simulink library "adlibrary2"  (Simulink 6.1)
undefined symbols (not defined in the file or in its folder): adlibrary2, ADM, Bit, Black, Box, d2sram_config, DDR, ddr32_config, ddr32xp_config, Generation, II, Inactive, Location, Lower, SDRAM, Simulation, Subsystem, Width, xbsIndex_r3, XPL, XRC, XRM, zbt32_config, zbt64_config, zbtXRC4_config
libraries: xbsIndex_r3 x786
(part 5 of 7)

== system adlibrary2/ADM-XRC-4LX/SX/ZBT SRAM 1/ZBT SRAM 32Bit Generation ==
  d : Inport  Port=1  LatchInput=off
  a : Inport  Port=2  LatchInput=off
  w : Inport  Port=3  LatchInput=off
  r : Inport  Port=4  LatchInput=off
  be : Inport  Port=5  LatchInput=off
  adlocb_in : Inport  Port=6  LatchInput=off
  Black Box : S-Function  FunctionName=xlblackbox2  Parameters=sfcn_mwsv__  mask(Xilinx Blackbox Block){init_code=zbtXRC4_config, sim_method=Inactive, engine_block=, show_param=on, xl_area=[88, 129, 0, 35, 0, 0, 0], xl_use_area=on, adlocb_devid=1}
      mask prompts: init_code "Block Configuration M-Function"; sim_method "Simulation Mode"; engine_block "HDL Co-Simulator To Use  (specify helper block by name)"; show_param "---------------------- Show Implementation Parameters -----------------------------------------------------------------------------------"; xl_area "FPGA Area [Slices, FFs, BRAMs, LUTs, IOBs, Emb. Mults, TBUFs]"; xl_use_area "Use Area Above For Estimation"; adlocb_devid "ADLOCB DEV ID"
      mask help: Incorporates black box HDL and simulation model into a System Generator design. You must supply a Black Box with certain information about the HDL component you would like to bring into System Generator. This information is provided through a Matlab function. When "Simulation Mode" is set to "Inactive," you will typically want to provide a separate simulation model by using a Simulation Multiplexer. When "Simulation Mode" is set to "Use HDL Co-Simulation", you must include a ModelSim block in the design.
      mask init:
      | [designRoot, family, part, speed, package, simulinkPeriod, sysclkPeriod, dbl_ovrd, trimVbit] = xlSysgenSettings(gcb,0,0);
      | 
      | [bg,fg] = xlcmap('XBlock');
      | iPos = get_param(gcb,'Position');
      | iWidth=iPos(3)-iPos(1); iHeight=iPos(4)-iPos(2);
      | iCx=iWidth/2;
      | iCy=iHeight/2;
      | [logoX, logoY] = xlogo(iPos);
      | zstr='z'; zpstr='-1';
      | zstrx = iCx-3; if (zstrx<16) zstr='';zpstr=''; end
      | zstry = iCy;
      | 
      | precision0 = 1;
      | latency = 0;
      | dblOvrd = 0;
      | 
      | mdlPath = xlGetMdlDir(bdroot);
      | 
      | refBlk = get_param(gcb,'referenceBlock');
      | if (isempty(refBlk) | strncmp(refBlk,'xbsIndex',8))
      | 	srcPath = mdlPath;
      | else
      | 	srcPath = xlPathToReference;
      | 	if (isempty(srcPath))
      | 		srcPath = mdlPath;
      | 	end
      | end
      | 
      | if (sim_method==2)
      | 	validEngineBlock = 0;
      | 	try
      | 	  engineBlock = xlBlockNameRelPath(get_param(gcb,'Parent'),engine_block);
      | 	catch
      | 	  engineBlock = '//';
      | 	end
      | 	try 
      | 	  engineWorkDir = get_param(engineBlock,'dir');
      | 	  validEngineBlock = 1;
      | 	catch
      | 	end
      | end
      | 
      | % just pass everything to s-function
      | sfcn_mwsv__ = get_param(gcb, 'MaskWSVariables');
      | adlocb_devid = 1;
      | plabel = xlbbPortLabelStruct(gcb,init_code,mdlPath);
  Constant : Constant  Value=0
  Terminator{,1..3} (4 alike) : Terminator
  ra1 : xbsIndex_r3/Gateway Out  output_type=Double  nbits=8  bin_pt=6  arith_type=Boolean  quantization=Truncate  overflow=Wrap  hdl_port=on  timing_constraint=None  locs_specified=off  LOCs={}  needs_fixed_name=off  show_param=off
  rc1 : xbsIndex_r3/Gateway Out  output_type=Double  nbits=8  bin_pt=6  arith_type=Boolean  quantization=Truncate  overflow=Wrap  hdl_port=on  timing_constraint=None  locs_specified=off  LOCs={}  needs_fixed_name=off  show_param=off
  rd1_i : xbsIndex_r3/Gateway In  arith_type=Unsigned  n_bits=32  bin_pt=0  quantization=Truncate  overflow=Wrap  period=1  timing_constraint=None  locs_specified=off  LOCs={}  needs_fixed_name=off  dbl_ovrd=off  show_param=off
  rd1_o : xbsIndex_r3/Gateway Out  output_type=Double  nbits=8  bin_pt=6  arith_type=Boolean  quantization=Truncate  overflow=Wrap  hdl_port=on  timing_constraint=None  locs_specified=off  LOCs={}  needs_fixed_name=off  show_param=off
  rd1_t : xbsIndex_r3/Gateway Out  output_type=Double  nbits=8  bin_pt=6  arith_type=Boolean  quantization=Truncate  overflow=Wrap  hdl_port=on  timing_constraint=None  locs_specified=off  LOCs={}  needs_fixed_name=off  show_param=off
  q : Outport
  qv : Outport  Port=2
  adlocb_out : Outport  Port=3
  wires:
  Black Box/7 -> adlocb_out/1
  adlocb_in/1 -> Black Box/7
  be/1 -> Black Box/5
  rd1_i/1 -> Black Box/6
  d/1 -> Black Box/1
  Black Box/1 -> q/1
  Black Box/2 -> qv/1
  Constant/1 -> rd1_i/1
  rd1_o/1 -> Terminator/1
  rd1_t/1 -> Terminator1/1
  ra1/1 -> Terminator2/1
  rc1/1 -> Terminator3/1
  a/1 -> Black Box/2
  w/1 -> Black Box/3
  r/1 -> Black Box/4
  Black Box/3 -> rd1_o/1
  Black Box/4 -> rd1_t/1
  Black Box/5 -> ra1/1
  Black Box/6 -> rc1/1

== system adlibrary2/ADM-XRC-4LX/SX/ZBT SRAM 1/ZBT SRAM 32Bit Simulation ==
  d : Inport  Port=1  LatchInput=off
  a : Inport  Port=2  LatchInput=off
  w : Inport  Port=3  LatchInput=off
  r : Inport  Port=4  LatchInput=off
  be : Inport  Port=5  LatchInput=off
  Disregard Subsystem : xbsIndex_r3/Disregard Subsystem  Tag=discardX
  Gateway In6 : xbsIndex_r3/Gateway In  arith_type=Boolean  n_bits=1  bin_pt=0  quantization=Truncate  overflow=Wrap  period=1  timing_constraint=None  locs_specified=off  LOCs={}  needs_fixed_name=off  dbl_ovrd=on  show_param=off
  Gateway In7 : xbsIndex_r3/Gateway In  arith_type=Unsigned  n_bits=32  bin_pt=0  quantization=Truncate  overflow=Wrap  period=1  timing_constraint=None  locs_specified=off  LOCs={}  needs_fixed_name=off  dbl_ovrd=on  show_param=off
  Gateway Out{,1..4} (5 alike) : xbsIndex_r3/Gateway Out  output_type=Double  nbits=8  bin_pt=6  arith_type=Boolean  quantization=Truncate  overflow=Wrap  hdl_port=off  timing_constraint=None  locs_specified=off  LOCs={}  needs_fixed_name=off  show_param=off
  S-Function : S-Function  FunctionName=zbt32  Parameters=1
  q : Outport
  qv : Outport  Port=2
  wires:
  be/1 -> Gateway Out4/1
  Gateway Out4/1 -> S-Function/5
  d/1 -> Gateway Out/1
  a/1 -> Gateway Out1/1
  w/1 -> Gateway Out2/1
  r/1 -> Gateway Out3/1
  S-Function/1 -> Gateway In7/1
  Gateway Out/1 -> S-Function/1
  Gateway Out1/1 -> S-Function/2
  Gateway Out2/1 -> S-Function/3
  Gateway Out3/1 -> S-Function/4
  Gateway In6/1 -> qv/1
  Gateway In7/1 -> q/1
  S-Function/2 -> Gateway In6/1

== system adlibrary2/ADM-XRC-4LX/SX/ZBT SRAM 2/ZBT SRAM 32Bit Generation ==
  d : Inport  Port=1  LatchInput=off
  a : Inport  Port=2  LatchInput=off
  w : Inport  Port=3  LatchInput=off
  r : Inport  Port=4  LatchInput=off
  be : Inport  Port=5  LatchInput=off
  adlocb_in : Inport  Port=6  LatchInput=off
  Black Box : S-Function  FunctionName=xlblackbox2  Parameters=sfcn_mwsv__  mask(Xilinx Blackbox Block){init_code=zbtXRC4_config, sim_method=Inactive, engine_block=, show_param=on, xl_area=[88, 129, 0, 35, 0, 0, 0], xl_use_area=on, adlocb_devid=2}
      mask prompts: init_code "Block Configuration M-Function"; sim_method "Simulation Mode"; engine_block "HDL Co-Simulator To Use  (specify helper block by name)"; show_param "---------------------- Show Implementation Parameters -----------------------------------------------------------------------------------"; xl_area "FPGA Area [Slices, FFs, BRAMs, LUTs, IOBs, Emb. Mults, TBUFs]"; xl_use_area "Use Area Above For Estimation"; adlocb_devid "ADLOCB DEV ID"
      mask help: Incorporates black box HDL and simulation model into a System Generator design. You must supply a Black Box with certain information about the HDL component you would like to bring into System Generator. This information is provided through a Matlab function. When "Simulation Mode" is set to "Inactive," you will typically want to provide a separate simulation model by using a Simulation Multiplexer. When "Simulation Mode" is set to "Use HDL Co-Simulation", you must include a ModelSim block in the design.
      mask init:
      | [designRoot, family, part, speed, package, simulinkPeriod, sysclkPeriod, dbl_ovrd, trimVbit] = xlSysgenSettings(gcb,0,0);
      | 
      | [bg,fg] = xlcmap('XBlock');
      | iPos = get_param(gcb,'Position');
      | iWidth=iPos(3)-iPos(1); iHeight=iPos(4)-iPos(2);
      | iCx=iWidth/2;
      | iCy=iHeight/2;
      | [logoX, logoY] = xlogo(iPos);
      | zstr='z'; zpstr='-1';
      | zstrx = iCx-3; if (zstrx<16) zstr='';zpstr=''; end
      | zstry = iCy;
      | 
      | precision0 = 1;
      | latency = 0;
      | dblOvrd = 0;
      | 
      | mdlPath = xlGetMdlDir(bdroot);
      | 
      | refBlk = get_param(gcb,'referenceBlock');
      | if (isempty(refBlk) | strncmp(refBlk,'xbsIndex',8))
      | 	srcPath = mdlPath;
      | else
      | 	srcPath = xlPathToReference;
      | 	if (isempty(srcPath))
      | 		srcPath = mdlPath;
      | 	end
      | end
      | 
      | if (sim_method==2)
      | 	validEngineBlock = 0;
      | 	try
      | 	  engineBlock = xlBlockNameRelPath(get_param(gcb,'Parent'),engine_block);
      | 	catch
      | 	  engineBlock = '//';
      | 	end
      | 	try 
      | 	  engineWorkDir = get_param(engineBlock,'dir');
      | 	  validEngineBlock = 1;
      | 	catch
      | 	end
      | end
      | 
      | % just pass everything to s-function
      | sfcn_mwsv__ = get_param(gcb, 'MaskWSVariables');
      | 
      | plabel = xlbbPortLabelStruct(gcb,init_code,mdlPath);
  Constant : Constant  Value=0
  Terminator{,1..3} (4 alike) : Terminator
  ra2 : xbsIndex_r3/Gateway Out  output_type=Double  nbits=8  bin_pt=6  arith_type=Boolean  quantization=Truncate  overflow=Wrap  hdl_port=on  timing_constraint=None  locs_specified=off  LOCs={}  needs_fixed_name=off  show_param=off
  rc2 : xbsIndex_r3/Gateway Out  output_type=Double  nbits=8  bin_pt=6  arith_type=Boolean  quantization=Truncate  overflow=Wrap  hdl_port=on  timing_constraint=None  locs_specified=off  LOCs={}  needs_fixed_name=off  show_param=off
  rd2_i : xbsIndex_r3/Gateway In  arith_type=Unsigned  n_bits=32  bin_pt=0  quantization=Truncate  overflow=Wrap  period=1  timing_constraint=None  locs_specified=off  LOCs={}  needs_fixed_name=off  dbl_ovrd=off  show_param=off
  rd2_o : xbsIndex_r3/Gateway Out  output_type=Double  nbits=8  bin_pt=6  arith_type=Boolean  quantization=Truncate  overflow=Wrap  hdl_port=on  timing_constraint=None  locs_specified=off  LOCs={}  needs_fixed_name=off  show_param=off
  rd2_t : xbsIndex_r3/Gateway Out  output_type=Double  nbits=8  bin_pt=6  arith_type=Boolean  quantization=Truncate  overflow=Wrap  hdl_port=on  timing_constraint=None  locs_specified=off  LOCs={}  needs_fixed_name=off  show_param=off
  q : Outport
  qv : Outport  Port=2
  adlocb_out : Outport  Port=3
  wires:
  Black Box/7 -> adlocb_out/1
  adlocb_in/1 -> Black Box/7
  be/1 -> Black Box/5
  rd2_i/1 -> Black Box/6
  d/1 -> Black Box/1
  Black Box/1 -> q/1
  Black Box/2 -> qv/1
  Constant/1 -> rd2_i/1
  rd2_o/1 -> Terminator/1
  rd2_t/1 -> Terminator1/1
  ra2/1 -> Terminator2/1
  rc2/1 -> Terminator3/1
  a/1 -> Black Box/2
  w/1 -> Black Box/3
  r/1 -> Black Box/4
  Black Box/3 -> rd2_o/1
  Black Box/4 -> rd2_t/1
  Black Box/5 -> ra2/1
  Black Box/6 -> rc2/1

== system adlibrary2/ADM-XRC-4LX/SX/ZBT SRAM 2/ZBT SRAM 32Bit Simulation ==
  d : Inport  Port=1  LatchInput=off
  a : Inport  Port=2  LatchInput=off
  w : Inport  Port=3  LatchInput=off
  r : Inport  Port=4  LatchInput=off
  be : Inport  Port=5  LatchInput=off
  Disregard Subsystem : xbsIndex_r3/Disregard Subsystem  Tag=discardX
  Gateway In6 : xbsIndex_r3/Gateway In  arith_type=Boolean  n_bits=1  bin_pt=0  quantization=Truncate  overflow=Wrap  period=1  timing_constraint=None  locs_specified=off  LOCs={}  needs_fixed_name=off  dbl_ovrd=on  show_param=off
  Gateway In7 : xbsIndex_r3/Gateway In  arith_type=Unsigned  n_bits=32  bin_pt=0  quantization=Truncate  overflow=Wrap  period=1  timing_constraint=None  locs_specified=off  LOCs={}  needs_fixed_name=off  dbl_ovrd=on  show_param=off
  Gateway Out{,1..4} (5 alike) : xbsIndex_r3/Gateway Out  output_type=Double  nbits=8  bin_pt=6  arith_type=Boolean  quantization=Truncate  overflow=Wrap  hdl_port=off  timing_constraint=None  locs_specified=off  LOCs={}  needs_fixed_name=off  show_param=off
  S-Function : S-Function  FunctionName=zbt32  Parameters=2
  q : Outport
  qv : Outport  Port=2
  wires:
  be/1 -> Gateway Out4/1
  Gateway Out4/1 -> S-Function/5
  d/1 -> Gateway Out/1
  a/1 -> Gateway Out1/1
  w/1 -> Gateway Out2/1
  r/1 -> Gateway Out3/1
  S-Function/1 -> Gateway In7/1
  Gateway Out/1 -> S-Function/1
  Gateway Out1/1 -> S-Function/2
  Gateway Out2/1 -> S-Function/3
  Gateway Out3/1 -> S-Function/4
  Gateway In6/1 -> qv/1
  Gateway In7/1 -> q/1
  S-Function/2 -> Gateway In6/1

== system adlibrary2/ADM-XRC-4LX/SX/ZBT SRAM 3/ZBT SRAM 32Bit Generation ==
  d : Inport  Port=1  LatchInput=off
  a : Inport  Port=2  LatchInput=off
  w : Inport  Port=3  LatchInput=off
  r : Inport  Port=4  LatchInput=off
  be : Inport  Port=5  LatchInput=off
  adlocb_in : Inport  Port=6  LatchInput=off
  Black Box : S-Function  FunctionName=xlblackbox2  Parameters=sfcn_mwsv__  mask(Xilinx Blackbox Block){init_code=zbtXRC4_config, sim_method=Inactive, engine_block=, show_param=on, xl_area=[88, 129, 0, 35, 0, 0, 0], xl_use_area=on, adlocb_devid=3}
      mask prompts: init_code "Block Configuration M-Function"; sim_method "Simulation Mode"; engine_block "HDL Co-Simulator To Use  (specify helper block by name)"; show_param "---------------------- Show Implementation Parameters -----------------------------------------------------------------------------------"; xl_area "FPGA Area [Slices, FFs, BRAMs, LUTs, IOBs, Emb. Mults, TBUFs]"; xl_use_area "Use Area Above For Estimation"; adlocb_devid "ADLOCB DEV ID"
      mask help: Incorporates black box HDL and simulation model into a System Generator design. You must supply a Black Box with certain information about the HDL component you would like to bring into System Generator. This information is provided through a Matlab function. When "Simulation Mode" is set to "Inactive," you will typically want to provide a separate simulation model by using a Simulation Multiplexer. When "Simulation Mode" is set to "Use HDL Co-Simulation", you must include a ModelSim block in the design.
      mask init:
      | [designRoot, family, part, speed, package, simulinkPeriod, sysclkPeriod, dbl_ovrd, trimVbit] = xlSysgenSettings(gcb,0,0);
      | 
      | [bg,fg] = xlcmap('XBlock');
      | iPos = get_param(gcb,'Position');
      | iWidth=iPos(3)-iPos(1); iHeight=iPos(4)-iPos(2);
      | iCx=iWidth/2;
      | iCy=iHeight/2;
      | [logoX, logoY] = xlogo(iPos);
      | zstr='z'; zpstr='-1';
      | zstrx = iCx-3; if (zstrx<16) zstr='';zpstr=''; end
      | zstry = iCy;
      | 
      | precision0 = 1;
      | latency = 0;
      | dblOvrd = 0;
      | 
      | mdlPath = xlGetMdlDir(bdroot);
      | 
      | refBlk = get_param(gcb,'referenceBlock');
      | if (isempty(refBlk) | strncmp(refBlk,'xbsIndex',8))
      | 	srcPath = mdlPath;
      | else
      | 	srcPath = xlPathToReference;
      | 	if (isempty(srcPath))
      | 		srcPath = mdlPath;
      | 	end
      | end
      | 
      | if (sim_method==2)
      | 	validEngineBlock = 0;
      | 	try
      | 	  engineBlock = xlBlockNameRelPath(get_param(gcb,'Parent'),engine_block);
      | 	catch
      | 	  engineBlock = '//';
      | 	end
      | 	try 
      | 	  engineWorkDir = get_param(engineBlock,'dir');
      | 	  validEngineBlock = 1;
      | 	catch
      | 	end
      | end
      | 
      | % just pass everything to s-function
      | sfcn_mwsv__ = get_param(gcb, 'MaskWSVariables');
      | adlocb_devid = 1;
      | plabel = xlbbPortLabelStruct(gcb,init_code,mdlPath);
  Constant : Constant  Value=0
  Terminator{,1..3} (4 alike) : Terminator
  ra3 : xbsIndex_r3/Gateway Out  output_type=Double  nbits=8  bin_pt=6  arith_type=Boolean  quantization=Truncate  overflow=Wrap  hdl_port=on  timing_constraint=None  locs_specified=off  LOCs={}  needs_fixed_name=off  show_param=off
  rc3 : xbsIndex_r3/Gateway Out  output_type=Double  nbits=8  bin_pt=6  arith_type=Boolean  quantization=Truncate  overflow=Wrap  hdl_port=on  timing_constraint=None  locs_specified=off  LOCs={}  needs_fixed_name=off  show_param=off
  rd3_i : xbsIndex_r3/Gateway In  arith_type=Unsigned  n_bits=32  bin_pt=0  quantization=Truncate  overflow=Wrap  period=1  timing_constraint=None  locs_specified=off  LOCs={}  needs_fixed_name=off  dbl_ovrd=off  show_param=off
  rd3_o : xbsIndex_r3/Gateway Out  output_type=Double  nbits=8  bin_pt=6  arith_type=Boolean  quantization=Truncate  overflow=Wrap  hdl_port=on  timing_constraint=None  locs_specified=off  LOCs={}  needs_fixed_name=off  show_param=off
  rd3_t : xbsIndex_r3/Gateway Out  output_type=Double  nbits=8  bin_pt=6  arith_type=Boolean  quantization=Truncate  overflow=Wrap  hdl_port=on  timing_constraint=None  locs_specified=off  LOCs={}  needs_fixed_name=off  show_param=off
  q : Outport
  qv : Outport  Port=2
  adlocb_out : Outport  Port=3
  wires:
  Black Box/6 -> rc3/1
  Black Box/5 -> ra3/1
  Black Box/4 -> rd3_t/1
  Black Box/3 -> rd3_o/1
  r/1 -> Black Box/4
  w/1 -> Black Box/3
  a/1 -> Black Box/2
  rc3/1 -> Terminator3/1
  ra3/1 -> Terminator2/1
  rd3_t/1 -> Terminator1/1
  rd3_o/1 -> Terminator/1
  Constant/1 -> rd3_i/1
  Black Box/2 -> qv/1
  Black Box/1 -> q/1
  d/1 -> Black Box/1
  rd3_i/1 -> Black Box/6
  be/1 -> Black Box/5
  adlocb_in/1 -> Black Box/7
  Black Box/7 -> adlocb_out/1

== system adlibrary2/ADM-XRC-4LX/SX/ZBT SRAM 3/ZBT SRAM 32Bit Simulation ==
  d : Inport  Port=1  LatchInput=off
  a : Inport  Port=2  LatchInput=off
  w : Inport  Port=3  LatchInput=off
  r : Inport  Port=4  LatchInput=off
  be : Inport  Port=5  LatchInput=off
  Disregard Subsystem : xbsIndex_r3/Disregard Subsystem  Tag=discardX
  Gateway In6 : xbsIndex_r3/Gateway In  arith_type=Boolean  n_bits=1  bin_pt=0  quantization=Truncate  overflow=Wrap  period=1  timing_constraint=None  locs_specified=off  LOCs={}  needs_fixed_name=off  dbl_ovrd=on  show_param=off
  Gateway In7 : xbsIndex_r3/Gateway In  arith_type=Unsigned  n_bits=32  bin_pt=0  quantization=Truncate  overflow=Wrap  period=1  timing_constraint=None  locs_specified=off  LOCs={}  needs_fixed_name=off  dbl_ovrd=on  show_param=off
  Gateway Out{,1..4} (5 alike) : xbsIndex_r3/Gateway Out  output_type=Double  nbits=8  bin_pt=6  arith_type=Boolean  quantization=Truncate  overflow=Wrap  hdl_port=off  timing_constraint=None  locs_specified=off  LOCs={}  needs_fixed_name=off  show_param=off
  S-Function : S-Function  FunctionName=zbt32  Parameters=3
  q : Outport
  qv : Outport  Port=2
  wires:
  S-Function/2 -> Gateway In6/1
  Gateway In7/1 -> q/1
  Gateway In6/1 -> qv/1
  Gateway Out3/1 -> S-Function/4
  Gateway Out2/1 -> S-Function/3
  Gateway Out1/1 -> S-Function/2
  Gateway Out/1 -> S-Function/1
  S-Function/1 -> Gateway In7/1
  r/1 -> Gateway Out3/1
  w/1 -> Gateway Out2/1
  a/1 -> Gateway Out1/1
  d/1 -> Gateway Out/1
  Gateway Out4/1 -> S-Function/5
  be/1 -> Gateway Out4/1

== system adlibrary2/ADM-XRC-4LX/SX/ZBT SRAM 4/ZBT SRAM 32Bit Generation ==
  d : Inport  Port=1  LatchInput=off
  a : Inport  Port=2  LatchInput=off
  w : Inport  Port=3  LatchInput=off
  r : Inport  Port=4  LatchInput=off
  be : Inport  Port=5  LatchInput=off
  adlocb_in : Inport  Port=6  LatchInput=off
  Black Box : S-Function  FunctionName=xlblackbox2  Parameters=sfcn_mwsv__  mask(Xilinx Blackbox Block){init_code=zbtXRC4_config, sim_method=Inactive, engine_block=, show_param=on, xl_area=[88, 129, 0, 35, 0, 0, 0], xl_use_area=on, adlocb_devid=4}
      mask prompts: init_code "Block Configuration M-Function"; sim_method "Simulation Mode"; engine_block "HDL Co-Simulator To Use  (specify helper block by name)"; show_param "---------------------- Show Implementation Parameters -----------------------------------------------------------------------------------"; xl_area "FPGA Area [Slices, FFs, BRAMs, LUTs, IOBs, Emb. Mults, TBUFs]"; xl_use_area "Use Area Above For Estimation"; adlocb_devid "ADLOCB DEV ID"
      mask help: Incorporates black box HDL and simulation model into a System Generator design. You must supply a Black Box with certain information about the HDL component you would like to bring into System Generator. This information is provided through a Matlab function. When "Simulation Mode" is set to "Inactive," you will typically want to provide a separate simulation model by using a Simulation Multiplexer. When "Simulation Mode" is set to "Use HDL Co-Simulation", you must include a ModelSim block in the design.
      mask init:
      | [designRoot, family, part, speed, package, simulinkPeriod, sysclkPeriod, dbl_ovrd, trimVbit] = xlSysgenSettings(gcb,0,0);
      | 
      | [bg,fg] = xlcmap('XBlock');
      | iPos = get_param(gcb,'Position');
      | iWidth=iPos(3)-iPos(1); iHeight=iPos(4)-iPos(2);
      | iCx=iWidth/2;
      | iCy=iHeight/2;
      | [logoX, logoY] = xlogo(iPos);
      | zstr='z'; zpstr='-1';
      | zstrx = iCx-3; if (zstrx<16) zstr='';zpstr=''; end
      | zstry = iCy;
      | 
      | precision0 = 1;
      | latency = 0;
      | dblOvrd = 0;
      | 
      | mdlPath = xlGetMdlDir(bdroot);
      | 
      | refBlk = get_param(gcb,'referenceBlock');
      | if (isempty(refBlk) | strncmp(refBlk,'xbsIndex',8))
      | 	srcPath = mdlPath;
      | else
      | 	srcPath = xlPathToReference;
      | 	if (isempty(srcPath))
      | 		srcPath = mdlPath;
      | 	end
      | end
      | 
      | if (sim_method==2)
      | 	validEngineBlock = 0;
      | 	try
      | 	  engineBlock = xlBlockNameRelPath(get_param(gcb,'Parent'),engine_block);
      | 	catch
      | 	  engineBlock = '//';
      | 	end
      | 	try 
      | 	  engineWorkDir = get_param(engineBlock,'dir');
      | 	  validEngineBlock = 1;
      | 	catch
      | 	end
      | end
      | 
      | % just pass everything to s-function
      | sfcn_mwsv__ = get_param(gcb, 'MaskWSVariables');
      | 
      | plabel = xlbbPortLabelStruct(gcb,init_code,mdlPath);
  Constant : Constant  Value=0
  Terminator{,1..3} (4 alike) : Terminator
  ra4 : xbsIndex_r3/Gateway Out  output_type=Double  nbits=8  bin_pt=6  arith_type=Boolean  quantization=Truncate  overflow=Wrap  hdl_port=on  timing_constraint=None  locs_specified=off  LOCs={}  needs_fixed_name=off  show_param=off
  rc4 : xbsIndex_r3/Gateway Out  output_type=Double  nbits=8  bin_pt=6  arith_type=Boolean  quantization=Truncate  overflow=Wrap  hdl_port=on  timing_constraint=None  locs_specified=off  LOCs={}  needs_fixed_name=off  show_param=off
  rd4_i : xbsIndex_r3/Gateway In  arith_type=Unsigned  n_bits=32  bin_pt=0  quantization=Truncate  overflow=Wrap  period=1  timing_constraint=None  locs_specified=off  LOCs={}  needs_fixed_name=off  dbl_ovrd=off  show_param=off
  rd4_o : xbsIndex_r3/Gateway Out  output_type=Double  nbits=8  bin_pt=6  arith_type=Boolean  quantization=Truncate  overflow=Wrap  hdl_port=on  timing_constraint=None  locs_specified=off  LOCs={}  needs_fixed_name=off  show_param=off
  rd4_t : xbsIndex_r3/Gateway Out  output_type=Double  nbits=8  bin_pt=6  arith_type=Boolean  quantization=Truncate  overflow=Wrap  hdl_port=on  timing_constraint=None  locs_specified=off  LOCs={}  needs_fixed_name=off  show_param=off
  q : Outport
  qv : Outport  Port=2
  adlocb_out : Outport  Port=3
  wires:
  Black Box/7 -> adlocb_out/1
  adlocb_in/1 -> Black Box/7
  be/1 -> Black Box/5
  rd4_i/1 -> Black Box/6
  d/1 -> Black Box/1
  Black Box/1 -> q/1
  Black Box/2 -> qv/1
  Constant/1 -> rd4_i/1
  rd4_o/1 -> Terminator/1
  rd4_t/1 -> Terminator1/1
  ra4/1 -> Terminator2/1
  rc4/1 -> Terminator3/1
  a/1 -> Black Box/2
  w/1 -> Black Box/3
  r/1 -> Black Box/4
  Black Box/3 -> rd4_o/1
  Black Box/4 -> rd4_t/1
  Black Box/5 -> ra4/1
  Black Box/6 -> rc4/1

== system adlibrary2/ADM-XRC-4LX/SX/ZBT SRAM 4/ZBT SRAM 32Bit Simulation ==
  d : Inport  Port=1  LatchInput=off
  a : Inport  Port=2  LatchInput=off
  w : Inport  Port=3  LatchInput=off
  r : Inport  Port=4  LatchInput=off
  be : Inport  Port=5  LatchInput=off
  Disregard Subsystem : xbsIndex_r3/Disregard Subsystem  Tag=discardX
  Gateway In6 : xbsIndex_r3/Gateway In  arith_type=Boolean  n_bits=1  bin_pt=0  quantization=Truncate  overflow=Wrap  period=1  timing_constraint=None  locs_specified=off  LOCs={}  needs_fixed_name=off  dbl_ovrd=on  show_param=off
  Gateway In7 : xbsIndex_r3/Gateway In  arith_type=Unsigned  n_bits=32  bin_pt=0  quantization=Truncate  overflow=Wrap  period=1  timing_constraint=None  locs_specified=off  LOCs={}  needs_fixed_name=off  dbl_ovrd=on  show_param=off
  Gateway Out{,1..4} (5 alike) : xbsIndex_r3/Gateway Out  output_type=Double  nbits=8  bin_pt=6  arith_type=Boolean  quantization=Truncate  overflow=Wrap  hdl_port=off  timing_constraint=None  locs_specified=off  LOCs={}  needs_fixed_name=off  show_param=off
  S-Function : S-Function  FunctionName=zbt32  Parameters=4
  q : Outport
  qv : Outport  Port=2
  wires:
  be/1 -> Gateway Out4/1
  Gateway Out4/1 -> S-Function/5
  d/1 -> Gateway Out/1
  a/1 -> Gateway Out1/1
  w/1 -> Gateway Out2/1
  r/1 -> Gateway Out3/1
  S-Function/1 -> Gateway In7/1
  Gateway Out/1 -> S-Function/1
  Gateway Out1/1 -> S-Function/2
  Gateway Out2/1 -> S-Function/3
  Gateway Out3/1 -> S-Function/4
  Gateway In6/1 -> qv/1
  Gateway In7/1 -> q/1
  S-Function/2 -> Gateway In6/1

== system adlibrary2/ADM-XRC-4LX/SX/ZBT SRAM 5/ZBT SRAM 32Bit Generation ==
  d : Inport  Port=1  LatchInput=off
  a : Inport  Port=2  LatchInput=off
  w : Inport  Port=3  LatchInput=off
  r : Inport  Port=4  LatchInput=off
  be : Inport  Port=5  LatchInput=off
  adlocb_in : Inport  Port=6  LatchInput=off
  Black Box : S-Function  FunctionName=xlblackbox2  Parameters=sfcn_mwsv__  mask(Xilinx Blackbox Block){init_code=zbtXRC4_config, sim_method=Inactive, engine_block=, show_param=on, xl_area=[88, 129, 0, 35, 0, 0, 0], xl_use_area=on, adlocb_devid=5}
      mask prompts: init_code "Block Configuration M-Function"; sim_method "Simulation Mode"; engine_block "HDL Co-Simulator To Use  (specify helper block by name)"; show_param "---------------------- Show Implementation Parameters -----------------------------------------------------------------------------------"; xl_area "FPGA Area [Slices, FFs, BRAMs, LUTs, IOBs, Emb. Mults, TBUFs]"; xl_use_area "Use Area Above For Estimation"; adlocb_devid "ADLOCB DEV ID"
      mask help: Incorporates black box HDL and simulation model into a System Generator design. You must supply a Black Box with certain information about the HDL component you would like to bring into System Generator. This information is provided through a Matlab function. When "Simulation Mode" is set to "Inactive," you will typically want to provide a separate simulation model by using a Simulation Multiplexer. When "Simulation Mode" is set to "Use HDL Co-Simulation", you must include a ModelSim block in the design.
      mask init:
      | [designRoot, family, part, speed, package, simulinkPeriod, sysclkPeriod, dbl_ovrd, trimVbit] = xlSysgenSettings(gcb,0,0);
      | 
      | [bg,fg] = xlcmap('XBlock');
      | iPos = get_param(gcb,'Position');
      | iWidth=iPos(3)-iPos(1); iHeight=iPos(4)-iPos(2);
      | iCx=iWidth/2;
      | iCy=iHeight/2;
      | [logoX, logoY] = xlogo(iPos);
      | zstr='z'; zpstr='-1';
      | zstrx = iCx-3; if (zstrx<16) zstr='';zpstr=''; end
      | zstry = iCy;
      | 
      | precision0 = 1;
      | latency = 0;
      | dblOvrd = 0;
      | 
      | mdlPath = xlGetMdlDir(bdroot);
      | 
      | refBlk = get_param(gcb,'referenceBlock');
      | if (isempty(refBlk) | strncmp(refBlk,'xbsIndex',8))
      | 	srcPath = mdlPath;
      | else
      | 	srcPath = xlPathToReference;
      | 	if (isempty(srcPath))
      | 		srcPath = mdlPath;
      | 	end
      | end
      | 
      | if (sim_method==2)
      | 	validEngineBlock = 0;
      | 	try
      | 	  engineBlock = xlBlockNameRelPath(get_param(gcb,'Parent'),engine_block);
      | 	catch
      | 	  engineBlock = '//';
      | 	end
      | 	try 
      | 	  engineWorkDir = get_param(engineBlock,'dir');
      | 	  validEngineBlock = 1;
      | 	catch
      | 	end
      | end
      | 
      | % just pass everything to s-function
      | sfcn_mwsv__ = get_param(gcb, 'MaskWSVariables');
      | adlocb_devid = 1;
      | plabel = xlbbPortLabelStruct(gcb,init_code,mdlPath);
  Constant : Constant  Value=0
  Terminator{,1..3} (4 alike) : Terminator
  ra5 : xbsIndex_r3/Gateway Out  output_type=Double  nbits=8  bin_pt=6  arith_type=Boolean  quantization=Truncate  overflow=Wrap  hdl_port=on  timing_constraint=None  locs_specified=off  LOCs={}  needs_fixed_name=off  show_param=off
  rc5 : xbsIndex_r3/Gateway Out  output_type=Double  nbits=8  bin_pt=6  arith_type=Boolean  quantization=Truncate  overflow=Wrap  hdl_port=on  timing_constraint=None  locs_specified=off  LOCs={}  needs_fixed_name=off  show_param=off
  rd5_i : xbsIndex_r3/Gateway In  arith_type=Unsigned  n_bits=32  bin_pt=0  quantization=Truncate  overflow=Wrap  period=1  timing_constraint=None  locs_specified=off  LOCs={}  needs_fixed_name=off  dbl_ovrd=off  show_param=off
  rd5_o : xbsIndex_r3/Gateway Out  output_type=Double  nbits=8  bin_pt=6  arith_type=Boolean  quantization=Truncate  overflow=Wrap  hdl_port=on  timing_constraint=None  locs_specified=off  LOCs={}  needs_fixed_name=off  show_param=off
  rd5_t : xbsIndex_r3/Gateway Out  output_type=Double  nbits=8  bin_pt=6  arith_type=Boolean  quantization=Truncate  overflow=Wrap  hdl_port=on  timing_constraint=None  locs_specified=off  LOCs={}  needs_fixed_name=off  show_param=off
  q : Outport
  qv : Outport  Port=2
  adlocb_out : Outport  Port=3
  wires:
  Black Box/6 -> rc5/1
  Black Box/5 -> ra5/1
  Black Box/4 -> rd5_t/1
  Black Box/3 -> rd5_o/1
  r/1 -> Black Box/4
  w/1 -> Black Box/3
  a/1 -> Black Box/2
  rc5/1 -> Terminator3/1
  ra5/1 -> Terminator2/1
  rd5_t/1 -> Terminator1/1
  rd5_o/1 -> Terminator/1
  Constant/1 -> rd5_i/1
  Black Box/2 -> qv/1
  Black Box/1 -> q/1
  d/1 -> Black Box/1
  rd5_i/1 -> Black Box/6
  be/1 -> Black Box/5
  adlocb_in/1 -> Black Box/7
  Black Box/7 -> adlocb_out/1

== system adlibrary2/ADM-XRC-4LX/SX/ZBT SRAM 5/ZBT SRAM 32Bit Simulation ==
  d : Inport  Port=1  LatchInput=off
  a : Inport  Port=2  LatchInput=off
  w : Inport  Port=3  LatchInput=off
  r : Inport  Port=4  LatchInput=off
  be : Inport  Port=5  LatchInput=off
  Disregard Subsystem : xbsIndex_r3/Disregard Subsystem  Tag=discardX
  Gateway In6 : xbsIndex_r3/Gateway In  arith_type=Boolean  n_bits=1  bin_pt=0  quantization=Truncate  overflow=Wrap  period=1  timing_constraint=None  locs_specified=off  LOCs={}  needs_fixed_name=off  dbl_ovrd=on  show_param=off
  Gateway In7 : xbsIndex_r3/Gateway In  arith_type=Unsigned  n_bits=32  bin_pt=0  quantization=Truncate  overflow=Wrap  period=1  timing_constraint=None  locs_specified=off  LOCs={}  needs_fixed_name=off  dbl_ovrd=on  show_param=off
  Gateway Out{,1..4} (5 alike) : xbsIndex_r3/Gateway Out  output_type=Double  nbits=8  bin_pt=6  arith_type=Boolean  quantization=Truncate  overflow=Wrap  hdl_port=off  timing_constraint=None  locs_specified=off  LOCs={}  needs_fixed_name=off  show_param=off
  S-Function : S-Function  FunctionName=zbt32  Parameters=5
  q : Outport
  qv : Outport  Port=2
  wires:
  S-Function/2 -> Gateway In6/1
  Gateway In7/1 -> q/1
  Gateway In6/1 -> qv/1
  Gateway Out3/1 -> S-Function/4
  Gateway Out2/1 -> S-Function/3
  Gateway Out1/1 -> S-Function/2
  Gateway Out/1 -> S-Function/1
  S-Function/1 -> Gateway In7/1
  r/1 -> Gateway Out3/1
  w/1 -> Gateway Out2/1
  a/1 -> Gateway Out1/1
  d/1 -> Gateway Out/1
  Gateway Out4/1 -> S-Function/5
  be/1 -> Gateway Out4/1

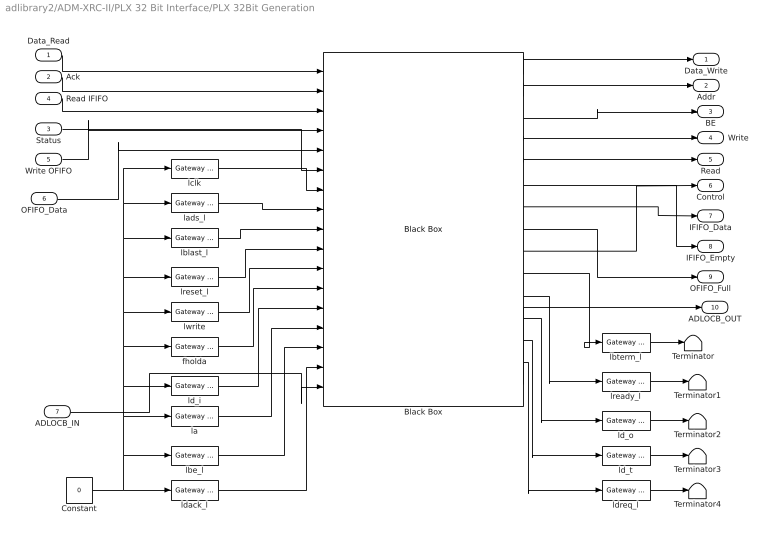
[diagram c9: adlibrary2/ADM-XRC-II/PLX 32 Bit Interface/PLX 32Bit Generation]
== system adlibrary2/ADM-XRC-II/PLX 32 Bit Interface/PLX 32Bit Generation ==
  Data_Read : Inport  Port=1  LatchInput=off
  Ack : Inport  Port=2  LatchInput=off
  Status : Inport  Port=3  LatchInput=off
  Read IFIFO : Inport  Port=4  LatchInput=off
  Write OFIFO : Inport  Port=5  LatchInput=off
  OFIFO_Data : Inport  Port=6  LatchInput=off
  ADLOCB_IN : Inport  Port=7  LatchInput=off
  Black Box : xbsIndex_r3/Black Box  init_code=lbif32_plx_config  sim_method=Inactive  show_param=on
  Constant : Constant  Value=0
  Terminator{,1..4} (5 alike) : Terminator
  fholda : xbsIndex_r3/Gateway In  arith_type=Boolean  n_bits=8  bin_pt=6  quantization=Truncate  overflow=Wrap  period=1  timing_constraint=None  locs_specified=off  LOCs={}  needs_fixed_name=off  dbl_ovrd=off  show_param=off
  la : xbsIndex_r3/Gateway In  arith_type=Unsigned  n_bits=24  bin_pt=0  quantization=Truncate  overflow=Wrap  period=1  timing_constraint=None  locs_specified=off  LOCs={}  needs_fixed_name=off  dbl_ovrd=off  show_param=off
  lads_l : xbsIndex_r3/Gateway In  arith_type=Boolean  n_bits=8  bin_pt=6  quantization=Truncate  overflow=Wrap  period=1  timing_constraint=None  locs_specified=off  LOCs={}  needs_fixed_name=off  dbl_ovrd=off  show_param=off
  lbe_l : xbsIndex_r3/Gateway In  arith_type=Unsigned  n_bits=4  bin_pt=0  quantization=Truncate  overflow=Wrap  period=1  timing_constraint=None  locs_specified=off  LOCs={}  needs_fixed_name=off  dbl_ovrd=off  show_param=off
  lblast_l : xbsIndex_r3/Gateway In  arith_type=Boolean  n_bits=8  bin_pt=6  quantization=Truncate  overflow=Wrap  period=1  timing_constraint=None  locs_specified=off  LOCs={}  needs_fixed_name=off  dbl_ovrd=off  show_param=off
  lbterm_l : xbsIndex_r3/Gateway Out  output_type=Double  nbits=8  bin_pt=6  arith_type=Boolean  quantization=Truncate  overflow=Wrap  hdl_port=on  timing_constraint=None  locs_specified=off  LOCs={}  needs_fixed_name=off  show_param=off
  lclk : xbsIndex_r3/Gateway In  arith_type=Boolean  n_bits=8  bin_pt=6  quantization=Truncate  overflow=Wrap  period=1  timing_constraint=None  locs_specified=off  LOCs={}  needs_fixed_name=off  dbl_ovrd=off  show_param=off
  ld_i : xbsIndex_r3/Gateway In  arith_type=Unsigned  n_bits=32  bin_pt=0  quantization=Truncate  overflow=Wrap  period=1  timing_constraint=None  locs_specified=off  LOCs={}  needs_fixed_name=off  dbl_ovrd=off  show_param=off
  ld_o : xbsIndex_r3/Gateway Out  output_type=Double  nbits=8  bin_pt=6  arith_type=Boolean  quantization=Truncate  overflow=Wrap  hdl_port=on  timing_constraint=None  locs_specified=off  LOCs={}  needs_fixed_name=off  show_param=off
  ld_t : xbsIndex_r3/Gateway Out  output_type=Double  nbits=8  bin_pt=6  arith_type=Boolean  quantization=Truncate  overflow=Wrap  hdl_port=on  timing_constraint=None  locs_specified=off  LOCs={}  needs_fixed_name=off  show_param=off
  ldack_l : xbsIndex_r3/Gateway In  arith_type=Unsigned  n_bits=2  bin_pt=0  quantization=Truncate  overflow=Wrap  period=1  timing_constraint=None  locs_specified=off  LOCs={}  needs_fixed_name=off  dbl_ovrd=off  show_param=off
  ldreq_l : xbsIndex_r3/Gateway Out  output_type=Double  nbits=8  bin_pt=6  arith_type=Boolean  quantization=Truncate  overflow=Wrap  hdl_port=on  timing_constraint=None  locs_specified=off  LOCs={}  needs_fixed_name=off  show_param=off
  lready_l : xbsIndex_r3/Gateway Out  output_type=Double  nbits=8  bin_pt=6  arith_type=Boolean  quantization=Truncate  overflow=Wrap  hdl_port=on  timing_constraint=None  locs_specified=off  LOCs={}  needs_fixed_name=off  show_param=off
  lreset_l : xbsIndex_r3/Gateway In  arith_type=Boolean  n_bits=8  bin_pt=6  quantization=Truncate  overflow=Wrap  period=1  timing_constraint=None  locs_specified=off  LOCs={}  needs_fixed_name=off  dbl_ovrd=off  show_param=off
  lwrite : xbsIndex_r3/Gateway In  arith_type=Boolean  n_bits=8  bin_pt=6  quantization=Truncate  overflow=Wrap  period=1  timing_constraint=None  locs_specified=off  LOCs={}  needs_fixed_name=off  dbl_ovrd=off  show_param=off
  Data_Write : Outport
  Addr : Outport  Port=2
  BE : Outport  Port=3
  Write : Outport  Port=4
  Read : Outport  Port=5
  Control : Outport  Port=6
  IFIFO_Data : Outport  Port=7
  IFIFO_Empty : Outport  Port=8
  OFIFO_Full : Outport  Port=9
  ADLOCB_OUT : Outport  Port=10
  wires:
  Data_Read/1 -> Black Box/1
  Write OFIFO/1 -> Black Box/4
  OFIFO_Data/1 -> Black Box/5
  lclk/1 -> Black Box/7
  lblast_l/1 -> Black Box/9
  lreset_l/1 -> Black Box/10
  lwrite/1 -> Black Box/11
  fholda/1 -> Black Box/12
  ld_i/1 -> Black Box/13
  la/1 -> Black Box/14
  lbe_l/1 -> Black Box/15
  ldack_l/1 -> Black Box/16
  Constant/1 -> ldack_l/1, lclk/1, lads_l/1, lblast_l/1, lreset_l/1, lwrite/1, fholda/1, ld_i/1, la/1, lbe_l/1
  lbterm_l/1 -> Terminator/1
  lready_l/1 -> Terminator1/1
  ld_o/1 -> Terminator2/1
  ld_t/1 -> Terminator3/1
  ldreq_l/1 -> Terminator4/1
  Black Box/1 -> Data_Write/1
  Black Box/2 -> Addr/1
  Black Box/3 -> BE/1
  Black Box/4 -> Write/1
  Black Box/5 -> Read/1
  Black Box/7 -> IFIFO_Data/1
  Black Box/8 -> OFIFO_Full/1
  Black Box/6 -> IFIFO_Empty/1
  Black Box/9 -> Control/1
  Black Box/10 -> lbterm_l/1
  Black Box/11 -> lready_l/1
  Black Box/12 -> ld_o/1
  Black Box/13 -> ld_t/1
  Black Box/14 -> ldreq_l/1
  Ack/1 -> Black Box/2
  Read IFIFO/1 -> Black Box/3
  lads_l/1 -> Black Box/8
  Status/1 -> Black Box/6
  ADLOCB_IN/1 -> Black Box/17
  Black Box/15 -> ADLOCB_OUT/1

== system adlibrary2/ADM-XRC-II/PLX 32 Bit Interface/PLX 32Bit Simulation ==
  Data_Read : Inport  Port=1  LatchInput=off
  Ack : Inport  Port=2  LatchInput=off
  Status : Inport  Port=3  LatchInput=off
  Read IFIFO : Inport  Port=4  LatchInput=off
  Write OFIFO : Inport  Port=5  LatchInput=off
  OFIFO_Data : Inport  Port=6  LatchInput=off
  Disregard Subsystem : xbsIndex_r3/Disregard Subsystem  Tag=discardX
  Gateway Out{,1..5} (6 alike) : xbsIndex_r3/Gateway Out  output_type=Double  nbits=8  bin_pt=6  arith_type=Boolean  quantization=Truncate  overflow=Wrap  hdl_port=off  timing_constraint=None  locs_specified=off  LOCs={}  needs_fixed_name=off  show_param=off
  S-Function : S-Function  FunctionName=lbif_plx32  Parameters=program,clock_ratio
  Subsystem : Subsystem
  Data_Write : Outport
  Addr : Outport  Port=2
  BE : Outport  Port=3
  Write : Outport  Port=4
  Read : Outport  Port=5
  Control : Outport  Port=6
  IFIFO_Data : Outport  Port=7
  IFIFO_Empty : Outport  Port=8
  OFIFO_Full : Outport  Port=9
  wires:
  Subsystem/2(Out2) -> Addr/1
  Subsystem/1(Out1) -> Data_Write/1
  S-Function/2 -> Subsystem/2(In2)
  S-Function/1 -> Subsystem/1(In1)
  Gateway Out5/1 -> S-Function/6
  Gateway Out4/1 -> S-Function/5
  Gateway Out3/1 -> S-Function/4
  Gateway Out2/1 -> S-Function/3
  Gateway Out1/1 -> S-Function/2
  Gateway Out/1 -> S-Function/1
  OFIFO_Data/1 -> Gateway Out5/1
  Write OFIFO/1 -> Gateway Out4/1
  Read IFIFO/1 -> Gateway Out3/1
  Status/1 -> Gateway Out2/1
  Ack/1 -> Gateway Out1/1
  Data_Read/1 -> Gateway Out/1
  S-Function/3 -> Subsystem/3(In9)
  Subsystem/3(Out9) -> BE/1
  S-Function/4 -> Subsystem/4(In3)
  S-Function/5 -> Subsystem/5(In4)
  S-Function/6 -> Subsystem/6(In5)
  S-Function/7 -> Subsystem/7(In6)
  S-Function/8 -> Subsystem/8(In7)
  S-Function/9 -> Subsystem/9(In8)
  Subsystem/4(Out3) -> Write/1
  Subsystem/5(Out4) -> Read/1
  Subsystem/6(Out5) -> Control/1
  Subsystem/7(Out6) -> IFIFO_Data/1
  Subsystem/8(Out7) -> IFIFO_Empty/1
  Subsystem/9(Out8) -> OFIFO_Full/1

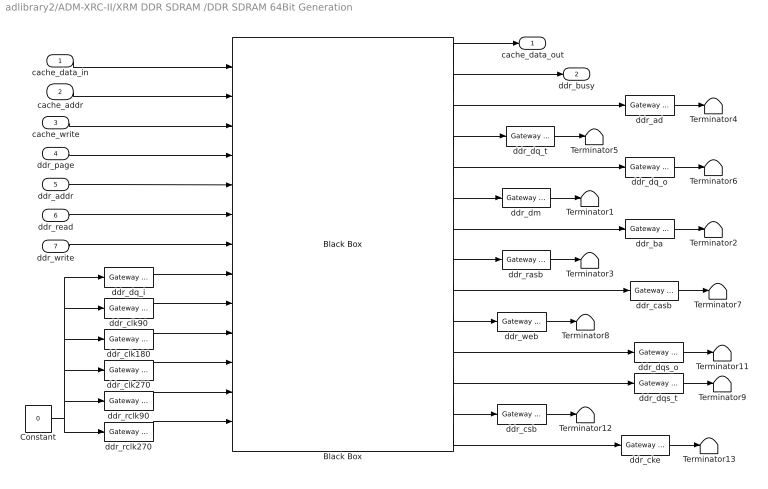
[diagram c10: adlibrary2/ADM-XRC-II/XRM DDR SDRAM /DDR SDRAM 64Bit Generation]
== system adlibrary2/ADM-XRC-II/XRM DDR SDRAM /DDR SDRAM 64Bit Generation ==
  cache_data_in : Inport  Port=1  LatchInput=off
  cache_addr : Inport  Port=2  LatchInput=off
  cache_write : Inport  Port=3  LatchInput=off
  ddr_page : Inport  Port=4  LatchInput=off
  ddr_addr : Inport  Port=5  LatchInput=off
  ddr_read : Inport  Port=6  LatchInput=off
  ddr_write : Inport  Port=7  LatchInput=off
  Black Box : xbsIndex_r3/Black Box  init_code=ddr64_config  sim_method=Inactive  show_param=on
  Constant : Constant  Value=0
  Terminator{1..9,11..13} (12 alike) : Terminator
  ddr_ad : xbsIndex_r3/Gateway Out  output_type=Double  nbits=8  bin_pt=6  arith_type=Boolean  quantization=Truncate  overflow=Wrap  hdl_port=on  timing_constraint=None  locs_specified=off  LOCs={}  needs_fixed_name=off  show_param=off
  ddr_ba : xbsIndex_r3/Gateway Out  output_type=Double  nbits=8  bin_pt=6  arith_type=Boolean  quantization=Truncate  overflow=Wrap  hdl_port=on  timing_constraint=None  locs_specified=off  LOCs={}  needs_fixed_name=off  show_param=off
  ddr_casb : xbsIndex_r3/Gateway Out  output_type=Double  nbits=8  bin_pt=6  arith_type=Boolean  quantization=Truncate  overflow=Wrap  hdl_port=on  timing_constraint=None  locs_specified=off  LOCs={}  needs_fixed_name=off  show_param=off
  ddr_cke : xbsIndex_r3/Gateway Out  output_type=Double  nbits=8  bin_pt=6  arith_type=Boolean  quantization=Truncate  overflow=Wrap  hdl_port=on  timing_constraint=None  locs_specified=off  LOCs={}  needs_fixed_name=off  show_param=off
  ddr_clk180 : xbsIndex_r3/Gateway In  arith_type=Boolean  n_bits=64  bin_pt=0  quantization=Truncate  overflow=Wrap  period=1  timing_constraint=None  locs_specified=off  LOCs={}  needs_fixed_name=off  dbl_ovrd=off  show_param=off
  ddr_clk270 : xbsIndex_r3/Gateway In  arith_type=Boolean  n_bits=64  bin_pt=0  quantization=Truncate  overflow=Wrap  period=1  timing_constraint=None  locs_specified=off  LOCs={}  needs_fixed_name=off  dbl_ovrd=off  show_param=off
  ddr_clk90 : xbsIndex_r3/Gateway In  arith_type=Boolean  n_bits=64  bin_pt=0  quantization=Truncate  overflow=Wrap  period=1  timing_constraint=None  locs_specified=off  LOCs={}  needs_fixed_name=off  dbl_ovrd=off  show_param=off
  ddr_csb : xbsIndex_r3/Gateway Out  output_type=Double  nbits=8  bin_pt=6  arith_type=Boolean  quantization=Truncate  overflow=Wrap  hdl_port=on  timing_constraint=None  locs_specified=off  LOCs={}  needs_fixed_name=off  show_param=off
  ddr_dm : xbsIndex_r3/Gateway Out  output_type=Double  nbits=8  bin_pt=6  arith_type=Boolean  quantization=Truncate  overflow=Wrap  hdl_port=on  timing_constraint=None  locs_specified=off  LOCs={}  needs_fixed_name=off  show_param=off
  ddr_dq_i : xbsIndex_r3/Gateway In  arith_type=Unsigned  n_bits=64  bin_pt=0  quantization=Truncate  overflow=Wrap  period=1  timing_constraint=None  locs_specified=off  LOCs={}  needs_fixed_name=off  dbl_ovrd=off  show_param=off
  ddr_dq_o : xbsIndex_r3/Gateway Out  output_type=Double  nbits=8  bin_pt=6  arith_type=Boolean  quantization=Truncate  overflow=Wrap  hdl_port=on  timing_constraint=None  locs_specified=off  LOCs={}  needs_fixed_name=off  show_param=off
  ddr_dq_t : xbsIndex_r3/Gateway Out  output_type=Double  nbits=8  bin_pt=6  arith_type=Boolean  quantization=Truncate  overflow=Wrap  hdl_port=on  timing_constraint=None  locs_specified=off  LOCs={}  needs_fixed_name=off  show_param=off
  ddr_dqs_o : xbsIndex_r3/Gateway Out  output_type=Double  nbits=8  bin_pt=6  arith_type=Boolean  quantization=Truncate  overflow=Wrap  hdl_port=on  timing_constraint=None  locs_specified=off  LOCs={}  needs_fixed_name=off  show_param=off
  ddr_dqs_t : xbsIndex_r3/Gateway Out  output_type=Double  nbits=8  bin_pt=6  arith_type=Boolean  quantization=Truncate  overflow=Wrap  hdl_port=on  timing_constraint=None  locs_specified=off  LOCs={}  needs_fixed_name=off  show_param=off
  ddr_rasb : xbsIndex_r3/Gateway Out  output_type=Double  nbits=8  bin_pt=6  arith_type=Boolean  quantization=Truncate  overflow=Wrap  hdl_port=on  timing_constraint=None  locs_specified=off  LOCs={}  needs_fixed_name=off  show_param=off
  ddr_rclk270 : xbsIndex_r3/Gateway In  arith_type=Boolean  n_bits=64  bin_pt=0  quantization=Truncate  overflow=Wrap  period=1  timing_constraint=None  locs_specified=off  LOCs={}  needs_fixed_name=off  dbl_ovrd=off  show_param=off
  ddr_rclk90 : xbsIndex_r3/Gateway In  arith_type=Boolean  n_bits=64  bin_pt=0  quantization=Truncate  overflow=Wrap  period=1  timing_constraint=None  locs_specified=off  LOCs={}  needs_fixed_name=off  dbl_ovrd=off  show_param=off
  ddr_web : xbsIndex_r3/Gateway Out  output_type=Double  nbits=8  bin_pt=6  arith_type=Boolean  quantization=Truncate  overflow=Wrap  hdl_port=on  timing_constraint=None  locs_specified=off  LOCs={}  needs_fixed_name=off  show_param=off
  cache_data_out : Outport
  ddr_busy : Outport  Port=2
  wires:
  Constant/1 -> ddr_clk90/1, ddr_dq_i/1, ddr_clk180/1, ddr_clk270/1, ddr_rclk90/1, ddr_rclk270/1
  ddr_clk90/1 -> Black Box/9
  ddr_dq_i/1 -> Black Box/8
  cache_data_in/1 -> Black Box/1
  cache_addr/1 -> Black Box/2
  cache_write/1 -> Black Box/3
  ddr_page/1 -> Black Box/4
  ddr_addr/1 -> Black Box/5
  ddr_read/1 -> Black Box/6
  ddr_write/1 -> Black Box/7
  Black Box/1 -> cache_data_out/1
  Black Box/2 -> ddr_busy/1
  ddr_ad/1 -> Terminator4/1
  ddr_dq_t/1 -> Terminator5/1
  ddr_dq_o/1 -> Terminator6/1
  ddr_dm/1 -> Terminator1/1
  ddr_ba/1 -> Terminator2/1
  ddr_rasb/1 -> Terminator3/1
  ddr_casb/1 -> Terminator7/1
  ddr_web/1 -> Terminator8/1
  ddr_dqs_o/1 -> Terminator11/1
  ddr_csb/1 -> Terminator12/1
  ddr_clk180/1 -> Black Box/10
  ddr_clk270/1 -> Black Box/11
  ddr_rclk90/1 -> Black Box/12
  ddr_rclk270/1 -> Black Box/13
  ddr_dqs_t/1 -> Terminator9/1
  ddr_cke/1 -> Terminator13/1
  Black Box/3 -> ddr_ad/1
  Black Box/4 -> ddr_dq_t/1
  Black Box/5 -> ddr_dq_o/1
  Black Box/6 -> ddr_dm/1
  Black Box/7 -> ddr_ba/1
  Black Box/8 -> ddr_rasb/1
  Black Box/9 -> ddr_casb/1
  Black Box/10 -> ddr_web/1
  Black Box/11 -> ddr_dqs_o/1
  Black Box/12 -> ddr_dqs_t/1
  Black Box/13 -> ddr_csb/1
  Black Box/14 -> ddr_cke/1

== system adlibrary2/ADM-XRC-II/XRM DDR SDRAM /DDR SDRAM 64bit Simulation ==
  cache_data_in : Inport  Port=1  LatchInput=off
  cache_addr : Inport  Port=2  LatchInput=off
  cache_write : Inport  Port=3  LatchInput=off
  ddr_page : Inport  Port=4  LatchInput=off
  ddr_addr : Inport  Port=5  LatchInput=off
  ddr_read : Inport  Port=6  LatchInput=off
  ddr_write : Inport  Port=7  LatchInput=off
  Disregard Subsystem : xbsIndex_r3/Disregard Subsystem  Tag=discardX
  S-Function : S-Function  FunctionName=ddr64  Parameters=memsize,0
  Subsystem : Subsystem
  gi{0..6} (7 alike) : xbsIndex_r3/Gateway Out  output_type=Double  nbits=8  bin_pt=6  arith_type=Boolean  quantization=Truncate  overflow=Wrap  hdl_port=off  timing_constraint=None  locs_specified=off  LOCs={}  needs_fixed_name=off  show_param=off
  cache_data_out : Outport
  ddr_busy : Outport  Port=2
  ddr_status : Outport  Port=3
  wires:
  S-Function/1 -> Subsystem/1(In1)
  S-Function/2 -> Subsystem/2(In2)
  cache_data_in/1 -> gi0/1
  cache_addr/1 -> gi1/1
  cache_write/1 -> gi2/1
  ddr_page/1 -> gi3/1
  ddr_addr/1 -> gi4/1
  ddr_read/1 -> gi5/1
  ddr_write/1 -> gi6/1
  gi0/1 -> S-Function/1
  gi1/1 -> S-Function/2
  gi2/1 -> S-Function/3
  gi3/1 -> S-Function/4
  gi4/1 -> S-Function/5
  gi5/1 -> S-Function/6
  gi6/1 -> S-Function/7
  S-Function/3 -> Subsystem/3(In3)
  Subsystem/1(Out1) -> cache_data_out/1
  Subsystem/2(Out2) -> ddr_busy/1
  Subsystem/3(Out3) -> ddr_status/1
